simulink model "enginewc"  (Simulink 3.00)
settings: Solver=ode23s  SolverMode=SingleTasking  StartTime=0.0  StopTime=10  RelTol=1e-3  AbsTol=1e-6
PreLoadFcn:
  | Kp=0.0614;Ki=0.0723;

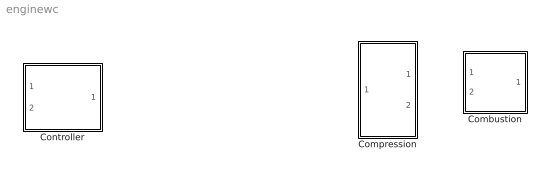
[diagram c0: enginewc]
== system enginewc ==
  Combustion : Subsystem
  Compression : Subsystem
  Controller : Subsystem

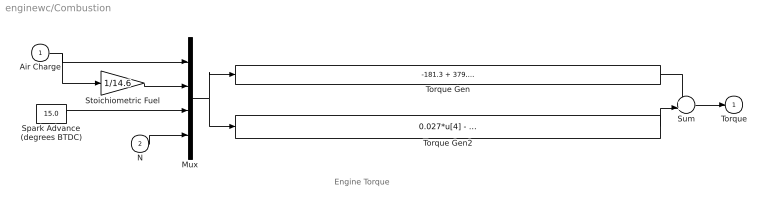
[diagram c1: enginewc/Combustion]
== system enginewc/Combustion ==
  note: Engine Torque
  Air Charge : Inport  Port=1  PortWidth=-1  SampleTime=-1  DataType=auto
  N : Inport  Port=2  PortWidth=-1  SampleTime=-1  DataType=auto
  Mux : Mux  Inputs=4
  Spark Advance (degrees BTDC) : Constant  Value=15.0
  Stoichiometric Fuel : Gain  Gain=1/14.6  SaturateOnIntegerOverflow=on
  Sum : Sum  Inputs=++  SaturateOnIntegerOverflow=on
  Torque Gen : Fcn  Expr=-181.3 + 379.36*u[1] + 21.91*u[1]/u[2] - (0.85*u[1]*u[1])/(u[2]*u[2]) + 0.26*u[3] - 0.0028*u[3]*u[3]
  Torque Gen2 : Fcn  Expr=0.027*u[4] - 0.000107*u[4]*u[4] + 0.00048*u[4]*u[3] + 2.55*u[3]*u[1] - 0.05*u[3]*u[3]*u[1]
  Torque : Outport  Port=1  InitialOutput=0
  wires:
  Stoichiometric Fuel/1 -> Mux/2
  Spark Advance (degrees BTDC)/1 -> Mux/3
  N/1 -> Mux/4
  Air Charge/1 -> Stoichiometric Fuel/1, Mux/1
  Mux/1 -> Torque Gen/1, Torque Gen2/1
  Torque Gen2/1 -> Sum/2
  Torque Gen/1 -> Sum/1
  Sum/1 -> Torque/1

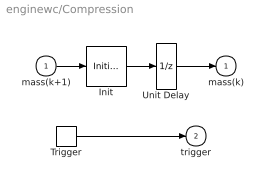
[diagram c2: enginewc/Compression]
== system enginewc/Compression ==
  mass(k+1) : Inport  Port=1  PortWidth=-1  SampleTime=-1  DataType=auto
  Trigger : TriggerPort  TriggerType=either  ShowOutputPort=on  OutputDataType=auto
  Init : InitialCondition  Value=0.152
  Unit Delay : UnitDelay  X0=0.152  SampleTime=-1
  mass(k) : Outport  Port=1  InitialOutput=0.152
  trigger : Outport  Port=2  InitialOutput=-1
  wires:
  Init/1 -> Unit Delay/1
  mass(k+1)/1 -> Init/1
  Unit Delay/1 -> mass(k)/1
  Trigger/1 -> trigger/1

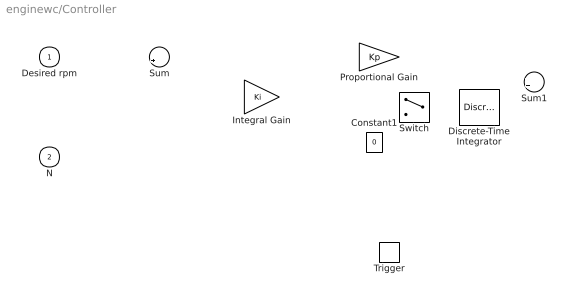
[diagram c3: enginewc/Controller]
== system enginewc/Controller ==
  Desired rpm : Inport  Port=1  PortWidth=-1  SampleTime=-1  DataType=auto
  N : Inport  Port=2  PortWidth=-1  SampleTime=-1  DataType=auto
  Trigger : TriggerPort  TriggerType=either  OutputDataType=auto
  Constant1 : Constant  Orientation=up  Value=0
  Discrete-Time Integrator : DiscreteIntegrator  IntegratorMethod=ForwardEuler  ExternalReset=none  InitialConditionSource=internal  InitialCondition=8.973  LimitOutput=off  UpperSaturationLimit=inf  LowerSaturationLimit=-inf  ShowSaturationPort=off  ShowStatePort=off  SampleTime=-1
  Integral Gain : Gain  Gain=Ki  SaturateOnIntegerOverflow=on
  Proportional Gain : Gain  Gain=Kp  SaturateOnIntegerOverflow=on
  Sum : Sum  Inputs=|+-  SaturateOnIntegerOverflow=on
  Sum1 : Sum  Inputs=++  SaturateOnIntegerOverflow=on
  Switch : Switch  T="\u0000 \u0000 \u0000 \u0000 \u0000 \u0000 \u0000 \u0000 \u0000 \u0000 \u0000 \u0000 \u0000 \u0000 \u0000 \u0000 \u0000 \u0000 \u0000 \u0000 \u0000 \u0000 \u0000 \u0000 \u0000 \u0000 \u0000 \u0000 \u0000 \u0000 \u0000 \u0000 \u0000 \u0000 \u0000 \u0000 \u0000 \u0000 \u0000 \u0000\u000e\u0000\u0000\u00008\u0000\u0000\u0000\u0006\u0000\u0000\u0000\b\u0000\u0000\u0000\u0004\u0000\u0000\u0000\u0000\u0000\u0000\u0000\u0005\u0000\u0000\u0000\b\u0000\u0000\u0000\u0001\u0000\u0000\u0000\u0003\u0000\u0000\u0000\u0001\u0000\u0000\u0000\u0000\u0000\u0000\u0000\u0004\u0000\u0000\u0000\u0006\u0000\u0000\u0000o\u0000f\u0000f\u0000\u0000\u0000\u000e\u0000\u0000\u00008\u0000\u0000\u0000\u0006\u0000\u0000\u0000\b\u0000\u0000\u0000\u0004\u0000\u0000\u0000\u0000\u0000\u0000\u0000\u0005\u0000\u0000\u0000\b\u0000\u0000\u0000\u0001\u0000\u0000\u0000\u0003\u0000\u0000\u0000\u0001\u0000\u0000\u0000\u0000\u0000\u0000\u0000\u0004\u0000\u0000\u0000\u0006\u0000\u0000\u0000o\u0000f\u0000f\u0000\u0000\u0000\u000e\u0000\u0000\u0000X\u0000\u0000\u0000\u0006\u0000\u0000\u0000\b\u0000\u0000\u0000\u0004\u0000\u0000\u0000\u0000\u0000\u0000\u0000\u0005\u0000\u0000\u0000\b\u0000\u0000\u0000\u0001\u0000\u0000\u0000\u0011\u0000\u0000\u0000\u0001\u0000\u0000\u0000\u0000\u0000\u0000\u0000\u0004\u0000\u0000\u0000\"\u0000\u0000\u0000P\u0000r\u0000i\u0000n\u0000t\u0000 \u0000P\u0000r\u0000e\u0000&\u0000v\u0000i\u0000e\u0000w\u0000.\u0000.\u0000.\u0000\u0000\u0000\u0000\u0000\u0000\u0000\u000e\u0000\u0000\u00008\u0000\u0000\u0000\u0006\u0000\u0000\u0000\b\u0000\u0000\u0000\u0004\u0000\u0000\u0000\u0000\u0000\u0000\u0000\u0005\u0000\u0000\u0000\b\u0000\u0000\u0000\u0001\u0000\u0000\u0000\u0003\u0000\u0000\u0000\u0001\u0000\u0000\u0000\u0000\u0000\u0000\u0000\u0004\u0000\u0000\u0000\u0006\u0000\u0000\u0000o\u0000f\u0000f\u0000\u0000\u0000\u000e\u0000\u0000\u0000`\u0000\u0000\u0000\u0006\u0000\u0000\u0000\b\u0000\u0000\u0000\u0004\u0000\u0000\u0000\u0000\u0000\u0000\u0000\u0005\u0000\u0000\u0000\b\u0000\u0000\u0000\u0001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"
